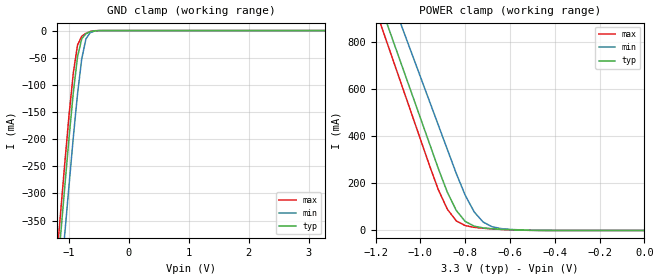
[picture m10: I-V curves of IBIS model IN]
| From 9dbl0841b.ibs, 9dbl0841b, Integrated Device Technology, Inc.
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|   Model IN
[Model]   IN
Model_type   Input
Polarity   Non-Inverting
Enable   Active-High
Vinl =   0.8000V
Vinh =   2.0000V
C_comp   1.1000pF   1.0000pF   1.2000pF
[Temperature Range]   25.0000   85.0000   -40.0
[Voltage Range]   3.3000V   3.0000V   3.6000V
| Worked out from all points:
|   GND clamp passes 1 mA (typ) near -0.59 V on its own axis
|   POWER clamp passes 1 mA (typ) near -0.52 V on its own axis
[GND_clamp]
|Voltage   I(typ)   I(min)   I(max)
-3.3V     -3.17A     -3.193A    -3.159A
-1.2V     -464.7mA   -547.4mA   -423.6mA
-1.13V    -374.6mA   -459.4mA   -332.5mA
-1.06V    -284.6mA   -371.3mA   -241.5mA
-990mV    -195.7mA   -283.2mA   -154.3mA
-920mV    -114mA     -196.3mA   -77.75mA
-850mV    -48.54mA   -116.7mA   -26.71mA
-780mV    -15.12mA   -52.18mA   -10.57mA
-710mV    -5.86mA    -15.39mA   -5.108mA
-640mV    -2.141mA   -3.955mA   -1.776mA
-500mV    -64.71uA   -173uA     -36.42uA
3.28V     102.5pA    3.816uA    94.41pA
[POWER_clamp]
|Voltage   I(typ)   I(min)   I(max)
-3.28V    6.621A     6.518A     6.681A
-1.2V     1.017A     1.168A     940.3mA
-1.16V    909.8mA    1.065A     829.9mA
-1.12V    802.1mA    962.8mA    719.6mA
-1.08V    694.4mA    860mA      609.3mA
-920mV    263.7mA    448.7mA    173.8mA
-880mV    163.5mA    345.8mA    90.98mA
-840mV    85.55mA    243.1mA    41.02mA
-800mV    38.57mA    150.2mA    20.78mA
-720mV    10.95mA    35.93mA    9.5mA
-600mV    3.201mA    4.59mA     2.795mA
0V        107.4pA    185.9pA    133.3pA
